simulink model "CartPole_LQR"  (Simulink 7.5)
settings: Solver=ode45  StartTime=0.0  StopTime=10.0  RelTol=1e-3
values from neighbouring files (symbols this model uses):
  g = 9.81    [Esercitazione09.m]
  K = lqrd(A,B,Q,R,Ts)    [Esercitazione09.m]
  L = 1    [Esercitazione09.m]
  m = 0.1    [Esercitazione09.m]
  M = 1    [Esercitazione09.m]
  ue = 0    [Esercitazione09.m]
  X0 = [1 0 0.55 0]'    [Esercitazione09.m]
  Xe = [1 0 0 0]'    [Esercitazione09.m]

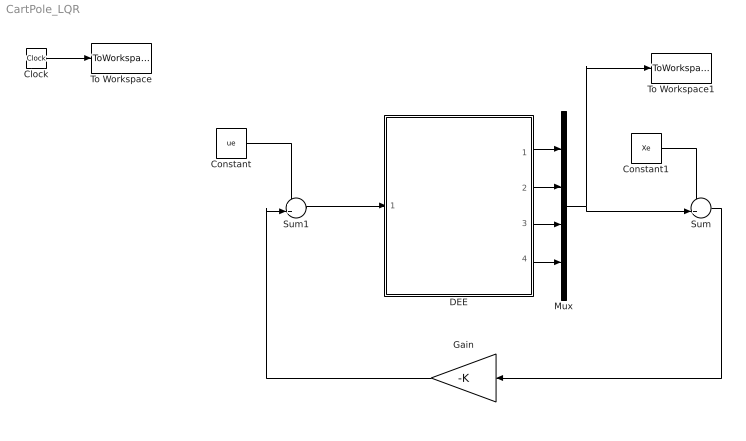
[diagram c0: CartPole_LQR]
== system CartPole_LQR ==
  Clock : Clock
  Constant : Constant  Value=ue  OutDataType=fixdt(1, 16)  OutScaling=2^0
  Constant1 : Constant  Value=Xe  OutDataType=fixdt(1, 16)  OutScaling=2^0
  DEE : Subsystem
  Gain : Gain  Gain=-K  Multiplication=Matrix(K*u)  ParameterDataType=fixdt(1, 16)  ParameterScaling=2^0  OutDataType=fixdt(1, 16)  OutScaling=2^0
  Mux : Mux
  Sum : Sum  Inputs=-+|  OutDataType=fixdt(1, 16)  OutScaling=2^0
  Sum1 : Sum  Inputs=++|  OutDataType=fixdt(1, 16)  OutScaling=2^0
  To Workspace : ToWorkspace  VariableName=time  SampleTime=-1  SaveFormat=Array
  To Workspace1 : ToWorkspace  VariableName=X  SampleTime=-1  SaveFormat=Array
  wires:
  DEE/1(Port1) -> Mux/1
  DEE/2(Port2) -> Mux/2
  DEE/4(Port4) -> Mux/4
  Clock/1 -> To Workspace/1
  DEE/3(Port3) -> Mux/3
  Mux/1 -> Sum/2, To Workspace1/1
  Sum/1 -> Gain/1
  Gain/1 -> Sum1/2
  Sum1/1 -> DEE/1(SysInport1)
  Constant/1 -> Sum1/1
  Constant1/1 -> Sum/1

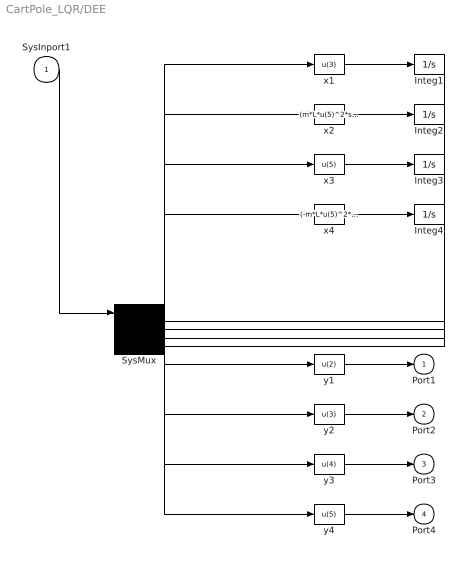
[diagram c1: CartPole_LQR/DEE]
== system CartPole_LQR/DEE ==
  SysInport1 : Inport
  Integ1 : Integrator  InitialCondition=X0(1)
  Integ2 : Integrator  InitialCondition=X0(2)
  Integ3 : Integrator  InitialCondition=X0(3)
  Integ4 : Integrator  InitialCondition=X0(4)
  SysMux : Mux  Inputs=5
  x1 : Fcn  Expr=u(3)
  x2 : Fcn  Expr=(m*L*u(5)^2*sin(u(4)) - m*g*sin(u(4))*cos(u(4))+ u)/(M+m*sin(u(4))^2)
  x3 : Fcn  Expr=u(5)
  x4 : Fcn  Expr=(-m*L*u(5)^2*sin(u(4))*cos(u(4))+(M+m)*g*sin(u(4))-u*cos(u(4)))/((M+m*sin(u(4))^2)*L)
  y1 : Fcn  Expr=u(2)
  y2 : Fcn  Expr=u(3)
  y3 : Fcn  Expr=u(4)
  y4 : Fcn  Expr=u(5)
  Port1 : Outport
  Port2 : Outport  Port=2
  Port3 : Outport  Port=3
  Port4 : Outport  Port=4
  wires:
  SysInport1/1 -> SysMux/1
  SysMux/1 -> x1/1, x2/1, x3/1, x4/1, y1/1, y2/1, y3/1, y4/1
  x1/1 -> Integ1/1
  Integ1/1 -> SysMux/2
  x2/1 -> Integ2/1
  Integ2/1 -> SysMux/3
  x3/1 -> Integ3/1
  Integ3/1 -> SysMux/4
  x4/1 -> Integ4/1
  Integ4/1 -> SysMux/5
  y1/1 -> Port1/1
  y2/1 -> Port2/1
  y3/1 -> Port3/1
  y4/1 -> Port4/1
